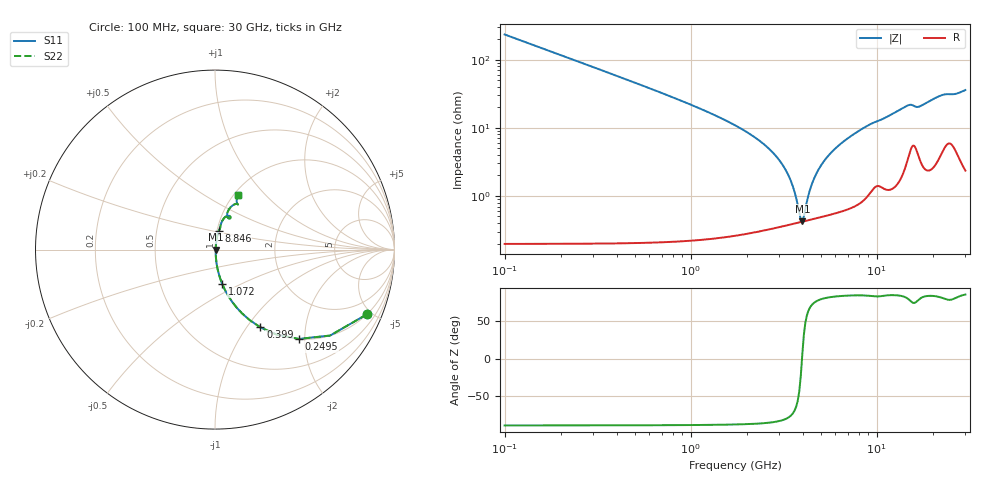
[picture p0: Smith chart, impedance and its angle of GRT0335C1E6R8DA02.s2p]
!Murata Part Number: GRT0335C1E6R8DA02
!These Parameters are Measured in Series Mode Connection
!Data Generated on Jun 19, 2026
!  o--ll--o
!Port1  Port2
!  o------o
!Operation Temp=25[degC], DC Bias Voltage=0[V]
!Freq. Start=100[MHz] Stop=30[GHz] 401[Steps]
# Hz S RI R 50
!Freq.(Hz) S11(Real) S11(Imag) S21(Real) S21(Imag) S12(Real) S12(Imag) S22(Real) S22(Imag)
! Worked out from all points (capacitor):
!   401 points, 100 MHz to 30 GHz, reference 50 ohm
!   read as one part in series: C = 6.8 pF near 249.5 MHz
!   lowest |Z| = 422 mohm at 3.987 GHz (marker M1)
!   series resonance near 3.971 GHz, so ESL is about 240 pH
!   S11 on the Smith chart (normalised r, x): 100 MHz: 1.00, -4.68; 249.5 MHz: 1.00, -1.87; 399 MHz: 1.00, -1.16; 1.072 GHz: 1.00, -0.40; 8.846 GHz: 1.02, +0.21; 30 GHz: 1.05, +0.71
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1e8  0.8453 -0.3612  0.1547 0.3612  0.1547 0.3612  0.8453 -0.3612
2.495e8  0.4661 -0.4978  0.5339 0.4978  0.5339 0.4978  0.4661 -0.4978
3.99e8  0.2528 -0.4329  0.7472 0.4329  0.7472 0.4329  0.2528 -0.4329
6.2325e8  0.1196 -0.3216  0.8804 0.3216  0.8804 0.3216  0.1196 -0.3216
1.07175e9  0.0412 -0.1934  0.9588 0.1934  0.9588 0.1934  0.0412 -0.1934
1.81925e9  0.0127 -0.0997  0.9873 0.0997  0.9873 0.0997  0.0127 -0.0997
3.01525e9  0.00454 -0.0323  0.9955 0.0323  0.9955 0.0323  0.00454 -0.0323
3.389e9  0.0041 -0.0184  0.9959 0.0184  0.9959 0.0184  0.0041 -0.0184
3.8375e9  0.00409 -0.00395  0.9959 0.00395  0.9959 0.00395  0.00409 -0.00395
3.987e9  0.00418 0.000473  0.9958 -0.000473  0.9958 -0.000473  0.00418 0.000473
4.06175e9  0.00424 0.00262  0.9958 -0.00262  0.9958 -0.00262  0.00424 0.00262
4.51025e9  0.00475 0.0147  0.9952 -0.0147  0.9952 -0.0147  0.00475 0.0147
5.10825e9  0.00579 0.0293  0.9942 -0.0293  0.9942 -0.0293  0.00579 0.0293
5.70625e9  0.00716 0.0426  0.9928 -0.0426  0.9928 -0.0426  0.00716 0.0426
6.5285e9  0.0095 0.0596  0.9905 -0.0596  0.9905 -0.0596  0.0095 0.0596
8.84575e9  0.0202 0.1022  0.9798 -0.1022  0.9798 -0.1022  0.0202 0.1022
1.01165e10  0.0285 0.1194  0.9715 -0.1194  0.9715 -0.1194  0.0285 0.1194
1.505e10  0.0795 0.1879  0.9205 -0.1879  0.9205 -0.1879  0.0795 0.1879
1.66945e10  0.0725 0.177  0.9275 -0.177  0.9275 -0.177  0.0725 0.177
2.005825e10  0.0845 0.2333  0.9155 -0.2333  0.9155 -0.2333  0.0845 0.2333
2.50665e10  0.1274 0.2517  0.8726 -0.2517  0.8726 -0.2517  0.1274 0.2517
3e10  0.1292 0.3041  0.8708 -0.3041  0.8708 -0.3041  0.1292 0.3041
